
FUNCTION_BLOCK FB6

TITLE =   <Control de arranque motor diesel>
//
//
//


AUTHOR:   H3       //  Hedgar Hernandez H.
FAMILY:   CAT      //  Caterpillar 3616
NAME:     C3616    //
VERSION:  01.01    //  Version Inicial 25/01/2009
// KNOW_HOW_PROTECT

//
//
//
//
//
//
//

VAR_INPUT

  MODO_REMOTO  : BOOL;	  // Selector en Modo remoto.
  ARRANQUE_REM : BOOL;    // Peticion de arranque remoto.
  PARO_REM     : BOOL;    // Peticion de paro remoto.
  REM_LISTO	   : BOOL;    // Condiciones para arranque en remoto ok.
  PARO_MAQUINA : BOOL;    // Paro de maquina por falla mayor.
  DIESEL_OP    : BOOL;    // Motor Diesel operando.
  POST_LUBE	   : BOOL;    // Postlubricacion Habilitada.
  TI_MARCHA    : TIME;    // Tiempo de marcha del motor.
  TI_POSTLUBE  : TIME;    // Tiempo de Postlubricacion.
  NUM_INTENTOS : INT;	  // Numero de intentos de arranque en modo automatico remoto.
  P_ARR_LISTA  : BOOL;    // Presion de prelubricacion lista.
  RESET        : BOOL;    // Reset de fallas.
  DIESEL_RPM   : REAL;    // Velocidad de la maquina diesel RPM.

END_VAR

VAR_OUTPUT
  VAL_ARRANQUE    : BOOL;	// Salida a valvula de Arranque.
  VAL_COMBUSTIBLE : BOOL;   // Valvula de corte de Combustible.
  VAL_AIRE        : BOOL; 	// Valvula de corte de Aire.
  BOMBA_PRELUB	  : BOOL;   // Bomba de prelubricacion.
  TORRETA		  : BOOL;   // Torreta para aviso de arranque.
  F_ARR_REM		  : BOOL;   // Falla de arranque remoto.
END_VAR

VAR
  TEMP1, TEMP2, TEMP3, TEMP4 : TON;
  paso : int;
  temp_ini_arranque : BOOL; 		// Bit auxiliar de secuencia de arranque
  f_arr_pres_lub : bool;			// Falla de arranque por falta de presion de lubricacion
  t_espera_prelub : time := T#1m;

END_VAR

// VAR_TEMP
//  ;
// END_VAR

BEGIN
NETWORK
TITLE =   <Inicializacion de secuencia de arranque remoto>
//
//

//Logica de inicializacion de secuencia de arranque remoto
//
		A MODO_REMOTO;
		A REM_LISTO;
		AN PARO_MAQUINA;
		AN DIESEL_OP;
		A ARRANQUE_REM;
		AN PARO_REM;
		S temp_ini_arranque;

		clr;
		O diesel_op;
		O paro_maquina;
		O Paro_rem;
		R temp_ini_arranque;


NETWORK
TITLE =   < Secuencia de lubricacion de arranque>
		//
		//
		A temp_ini_arranque;
		AN diesel_op;
		AN p_arr_lista;
		S bomba_prelub;

	//	call temp1
	//	   (in := bomba_prelub, pt:= t_espera_prelub);



NETWORK
TITLE =   < Secuencia de arranque>
//
//



NETWORK
TITLE =   < Secuencia de Paro>
//
//



NETWORK
TITLE =   < Secuencia de Postlubricacion>
//
//


END_FUNCTION_BLOCK


FUNCTION_BLOCK FB21

TITLE =   <interner Baustein-Titel/ Internal block title>
//
//   <Baustein-Kommentar/ Block comment>
//   Hier können Sie Informationen zu Ihrem Baustein hinterlegen
//   You can store information about your block here
//
//   statt FB<Baustein-Nr> kann auch <Name aus Symboltabelle> angegeben werden;
//   In place of FB<block no.>, <symbolic name> can also be entered;

AUTHOR:   Andy     //  max. 8 Zeichen / max. 8 characters
FAMILY:   plant1   //  max. 8 Zeichen / max. 8 characters
NAME:     fb_mot21 //  max. 8 Zeichen / max. 8 characters
VERSION:  01.01    //  max. 15.15
// KNOW_HOW_PROTECT
//   (falls angegeben, kann im generierten Baustein keine Änderungen mehr vorgenommen werden)
//   (If specified, no more changes can be made once the block is generated)
//
//   Die Vorbelegung von Variablen ist nur für INPUT-, OUTPUT-, IN_OUT-
//   und VAR- Variable möglich; nicht für VAR_TEMP.
//   Assigning variables is only possible for INPUT, OUTPUT, IN_OUT,
//   and VAR variables; not for VAR_TEMP

VAR_INPUT
  IN1: INT:=123;
END_VAR

VAR_OUTPUT
  OUT1: INT:=123;
END_VAR

VAR_IN_OUT
  IN_OUT1: INT:=123;
END_VAR

VAR
  VAR1: INT:=123;
END_VAR

VAR_TEMP
  TEMP1: INT;
END_VAR

BEGIN
NETWORK
TITLE =   <Überschrift von 1. Netzwerk/ Title of first network>
//
//  <Netzwerk-Kommentar/ Network comment>
//  Hier können Sie Informationen zu Ihrem Netzwerk hinterlegen
//  You can store information about your network here

//  Anweisungen des Netzwerks
//  z.B. FB-Aufruf:
//  CALL FB1, DB1
//    ( <Parameter-Name>:=<Aktualparameter>   ; weitere Parameter
//     );
//   Parameterübergaben sind beim FB optional, sie können einzeln oder gesamt
//   (incl. () ) weggelassen werden. Auch beim Aufruf kann statt FB bzw.
//   DB<Baustein-Nr> ein Name aus der Symboltabelle angegeben werden.

//  Instructions in the network
//  for example, FB call:
//  CALL FB1, DB1
//    ( <parameter name>:=<actual parameter>   ; additional parameters
//     );
//   Parameter passing is optional in the FB, individual parameters or the whole
//   parameter (including () ) can be left out. For the block call, you can also specify
//   a symbolic name from the symbol table instead of the FB or DB<block no.>.

//   Folge-Netzwerke/ Other networks


END_FUNCTION_BLOCK

